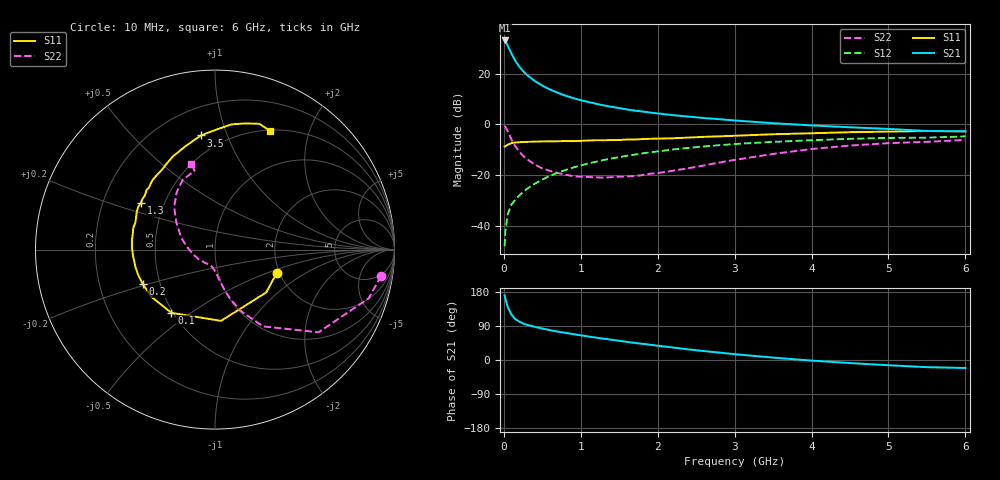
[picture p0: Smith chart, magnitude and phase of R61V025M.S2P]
! SIEMENS Small Signal Semiconductors
! BFR193
! Si NPN RF Bipolar Junction Transistor in SOT23
! VCE = 1 V  IC = 25 mA
! Common Emitter S-Parameters:  May  1996
# GHz  S  MA  R  50
!  f  S11  S21  S12  S22
! GHz  MAG  ANG  MAG  ANG  MAG  ANG  MAG  ANG
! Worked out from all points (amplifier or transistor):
!   36 points, 10 MHz to 6 GHz, reference 50 ohm
!   highest |S21| = 33.1 dB at 10 MHz (marker M1)
!   |S21| within 3 dB of that: start of sweep to 66.12 MHz
!   unconditionally stable (mu >= 1): 443.8 MHz to 2.216 GHz
!   at 250 MHz: K = 0.89, MSG = 23.8 dB, |S12| = -26.6 dB
!   at 1.4 GHz: K = 1.03, MAG = 9.1 dB, |S12| = -13.4 dB
!   at 6 GHz: K = 0.97, MSG = 1.0 dB, |S12| = -4.7 dB
!   S11 on the Smith chart (normalised r, x): 10 MHz: 1.93, -0.59; 100 MHz: 0.49, -0.42; 200 MHz: 0.40, -0.19; 1.3 GHz: 0.37, +0.25; 3.5 GHz: 0.38, +0.81; 6 GHz: 0.51, +1.44
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0.01  0.3676 -21.1  45.15 170.6  0.004 83.6  0.9368 -9.0
0.02  0.372 -39.9  43.89 161.4  0.0078 76.7  0.898 -17.6
0.05  0.3984 -85.2  36.21 139.9  0.0169 67.9  0.7385 -38.6
0.1  0.4282 -124.6  24.59 119.2  0.0265 60.4  0.5045 -58.0
0.15  0.4412 -143.3  17.86 107.9  0.0331 61.3  0.3701 -67.3
0.2  0.4461 -154.7  13.88 101.4  0.0398 63.5  0.2909 -72.5
0.25  0.4507 -162.0  11.25 96.5  0.0466 65.1  0.2404 -76.0
0.3  0.4538 -167.6  9.475 93.0  0.0538 66.8  0.2079 -78.3
0.4  0.458 -175.6  7.216 87.7  0.0677 68.5  0.1633 -82.6
0.5  0.463 178.7  5.804 83.0  0.0822 69.0  0.1359 -86.1
0.6  0.4658 173.7  4.872 78.8  0.0968 68.8  0.1215 -89.3
0.7  0.4666 169.1  4.206 74.9  0.1116 68.5  0.1109 -92.6
0.8  0.4711 165.1  3.696 71.6  0.1262 67.4  0.1025 -96.8
0.9  0.4687 161.1  3.31 68.3  0.1416 66.7  0.0958 -100.8
1.1  0.4827 154.8  2.763 62.0  0.1706 64.3  0.0922 -109.5
1.3  0.4885 147.7  2.372 56.2  0.1996 61.6  0.0894 -119.1
1.7  0.505 136.7  1.875 45.1  0.2548 56.0  0.0959 -141.2
2.2  0.5339 123.7  1.523 32.9  0.3208 48.1  0.1227 -166.1
3.5  0.6409 97.0  1.059 6.3  0.454 27.0  0.2624 145.1
4.5  0.7042 82.4  0.879 -8.1  0.5209 12.9  0.3838 123.8
5.5  0.743 70.6  0.743 -18.9  0.5495 -0.7  0.4545 104.4
6  0.7293 65.1  0.734 -21.1  0.5815 -4.7  0.4954 105.6
